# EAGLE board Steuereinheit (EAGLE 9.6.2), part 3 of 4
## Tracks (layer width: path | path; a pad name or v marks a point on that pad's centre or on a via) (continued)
N$83  (via drill 0.35) (continued)
  Top 0.152: v113.72,92.33 112.47,92.33 110.52,90.37 110.52,89.66 PC_JK6.4 | v136.12,95.17 136.12,94.64 137.9,92.86 140.03,92.86 142.16,95 142.16,95.71 PC_AN10.10
  Route2 0.152: v113.72,92.33 114.25,92.33 117.09,95.17 v136.12,95.17
N$84  (via drill 0.35)
  Top 0.152: v115.67,97.49 115.67,95.88 PC_JK6.9 | v115.67,114.02 132.56,114.02 134.16,112.42 134.16,100.86 136.83,98.2 139.68,98.2 140.92,96.95 140.92,95.88 PC_AN10.11
  Bottom 0.152: v115.67,114.02 v115.67,97.49
N$85  (via drill 0.35)
  Top 0.152: PC_JK6.12 111.76,94.64 113,93.4 117.8,93.4 v118.16,93.75 | v135.94,79.17 135.94,77.57 136.65,76.86 138.96,76.86 139.68,77.57 139.68,78.1 PC_AN11.3
  Route15 0.152: v118.16,93.75 122.25,93.75 126.16,89.84 128.65,89.84 135.94,82.55 v135.94,79.17
N$86  (via drill 0.35)
  Top 0.152: v118.16,77.04 117.98,76.86 114.96,76.86 114.43,77.39 114.43,78.1 PC_JK7.7 | v140.74,79.88 140.74,78.46 140.92,78.28 PC_AN11.4
  Route15 0.152: v118.16,77.04 121.72,77.04 122.78,78.1 138.96,78.1 v140.74,79.88
N$87  (via drill 0.35)
  Top 0.152: v122.25,83.97 118.52,83.97 116.38,81.84 112.29,81.84 110.52,80.06 110.52,78.28 PC_JK7.4 | v143.05,82.73 142.34,83.44 142.34,84.33 PC_AN11.10
  Route15 0.152: v122.25,83.97 128.65,83.97 134.16,78.46 136.47,78.46 140.03,82.02 142.34,82.02 v143.05,82.73
N$88  (via drill 0.35)
  Top 0.152: v146.43,96.06 145.01,97.49 143.76,97.49 142.16,99.09 142.16,101.04 PC_AN5.5 | v146.43,70.28 145.9,70.28 143.59,67.97 143.59,66.9 PC_NO1.6
  Bottom 0.152: v146.43,70.28 v146.43,96.06
N$89  (via drill 0.35)
  Top 0.152: v77.62,37.39 76.02,35.79 72.11,35.79 69.98,37.92 69.98,38.63 BR_NO2.14 | v77.27,50.55 76.38,50.55 75.49,51.44 73.18,51.44 72.47,50.72 72.47,50.19 BR_AN1.10 | v87.4,48.41 87.58,48.59 87.58,50.01 BR_JK1.10
  Route15 0.152: v87.4,48.41 86.69,49.12 78.69,49.12 v77.27,50.55
  Bottom 0.152: v77.62,37.39 77.62,40.59 77.98,40.95 77.98,49.84 v77.27,50.55
N$90
  Top 0.152: BR_OR2.4 57.17,66.9 57.17,69.75 59.66,72.24 59.66,72.77 BR_OR2.9
N$91  (via drill 0.35)
  Top 0.152: v125.09,88.06 124.21,88.06 123.32,88.95 123.32,89.48 PC_AN6.1 | v144.3,74.73 144.3,73.3 144.65,72.95 PC_NO1.10
  Route2 0.152: v125.09,88.06 126.34,88.06 126.69,88.42 129.72,88.42 142.7,75.44 143.59,75.44 v144.3,74.73
N$92
  Top 0.152: BR_OR2.3 55.93,66.73 55.93,66.02 58.24,63.7 60.38,63.7 61.62,64.95 61.62,72.24 61.09,72.77 BR_OR2.8
N$93  (via drill 0.35)
  Top 0.152: v135.94,93.22 133.45,95.71 130.96,95.71 PC_AN6.8 | v144.12,71.35 143.23,71.35 142.34,72.24 142.34,72.77 PC_NO1.12
  Route2 0.152: v135.94,93.22 138.61,93.22 139.14,92.69 140.03,92.69 145.36,87.35 145.36,72.59 v144.12,71.35
N$94  (via drill 0.35)
  Top 0.152: v35.84,43.43 33.88,41.48 31.04,41.48 29.26,43.26 29.26,43.79 BR_OR1.3 | v72.82,48.41 72.82,47.88 73.71,46.99 74.42,46.99 74.78,47.35 74.78,50.01 BR_AN1.8
  Route2 0.152: v35.84,43.43 35.84,44.68 42.06,50.9 60.73,50.9 63.22,48.41 v72.82,48.41
N$95
  Top 0.152: PC_NO1.15 138.43,73.48 136.83,75.08 130.78,75.08 130.43,75.44 127.23,75.44 127.05,75.62 125.09,75.62 123.32,77.39 123.32,78.1 PC_AN7.1
N$96  (via drill 0.35)
  Top 0.152: v83.67,20.14 83.67,18.54 BR_AN3.4 | v56.29,68.5 54.51,70.28 54.33,70.28 53.98,70.64 53.98,71.7 54.51,72.24 54.51,72.77 BR_OR2.13
  Route15 0.152: v83.67,20.14 83.67,20.68 72.82,31.52 70.69,31.52 61.09,41.12 57.71,41.12 v55.75,39.17
  Bottom 0.152: v55.75,39.17 55.22,39.7 55.22,67.44 v56.29,68.5
N$97  (via drill 0.35)
  Top 0.152: PC_NO2.2 138.43,54.63 137.72,53.92 136.65,53.92 v133.99,56.59 | v132.92,82.37 130.96,84.33 PC_AN7.8
  Bottom 0.152: v133.99,56.59 133.99,81.31 v132.92,82.37
N$98  (via drill 0.35)
  Top 0.152: v72.11,40.59 69.98,40.59 68.73,39.34 68.73,38.63 BR_NO2.15 | v86.33,48.41 86.33,50.01 BR_JK1.11
  Route2 0.152: v72.11,40.59 79.58,48.06 85.98,48.06 v86.33,48.41
N$99  (via drill 0.35)
  Top 0.152: v131.5,59.26 134.16,59.26 135.23,58.19 139.32,58.19 140.92,56.59 140.92,55.35 PC_NO2.4 | v125.27,64.77 124.56,64.77 123.32,66.02 123.32,66.73 PC_AN8.1
  Route2 0.152: v131.5,59.26 130.78,59.26 v125.27,64.77
N$100  (via drill 0.35)
  Top 0.152: BR_AN3.5 85.09,17.83 88.65,14.28 92.73,14.28 | 92.73,14.28 94.16,14.28 97.71,17.83 | 97.71,17.83 97.71,18.36 BR_AN4.5 97.71,17.83 | v92.73,15.34 92.73,18.36 BR_AN4.1 | 92.73,14.28 v92.73,13.92 | 97.71,17.83 98.42,17.12 100.91,17.12 101.09,17.3 101.09,19.96 100.38,20.68 100.38,24.59 BR_AN4.8 100.2,24.77 100.2,25.48 99.67,26.01 95.94,26.01 95.4,25.48 95.4,24.77 BR_AN4.12 95.4,24.59 95.4,23.52 95.58,23.34 95.58,22.63 95.05,22.1 93.09,22.1 91.14,24.05 87.58,24.05 | v80.64,20.14 80.11,19.61 80.11,18.54 BR_AN3.1 | v80.64,22.63 81.18,22.63 82.42,23.88 | 82.42,23.88 82.42,24.59 BR_AN3.12 82.42,23.88 | 87.58,24.05 87.58,24.59 BR_AN3.8 87.58,24.05 | 87.58,24.05 85.8,22.28 84.02,22.28 82.42,23.88 | v135.23,80.59 138.07,80.59 140.92,83.44 140.92,84.33 PC_AN11.11
  Route2 0.152: v135.23,80.59 134.7,80.59 126.16,72.06 124.21,72.06 109.8,57.66 109.27,57.66 92.56,40.95 92.56,37.92 92.02,37.39 92.02,35.61 84.56,28.14 84.56,26.19 81,22.63 v80.64,22.63
  Bottom 0.152: v92.73,13.92 v92.73,15.34 | v80.64,22.63 v80.64,20.14
N$101  (via drill 0.35)
  Top 0.152: v146.79,57.3 146.79,54.1 146.61,53.92 144.3,53.92 143.59,54.63 143.59,55.35 PC_NO2.6 | v144.3,69.75 133.99,69.75 PC_AN8.8
  Bottom 0.152: v146.79,57.3 144.3,59.79 v144.3,69.75
N$102  (via drill 0.35)
  Top 0.152: v79.22,26.19 77.8,27.61 71.58,27.61 70.87,26.9 70.16,26.9 68.73,25.48 68.73,24.77 BR_OR4.13 | v88.29,22.99 91.67,22.99 92.91,21.74 95.4,21.74 96.47,22.81 96.47,24.59 BR_AN4.11
  Route2 0.152: v88.29,22.99 v85.45,22.99
  Route15 0.152: v79.22,26.19 81.36,26.19 84.56,22.99 v85.45,22.99
N$103  (via drill 0.35)
  Top 0.152: v149.28,91.62 150.17,90.73 150.17,68.33 144.83,62.99 144.83,61.57 PC_NO2.10 | v122.25,100.51 122.61,100.51 123.14,101.04 PC_AN9.1
  Route2 0.152: v149.28,91.62 146.25,91.62 144.65,93.22 139.14,93.22 131.85,100.51 v122.25,100.51
N$104  (via drill 0.35)
  Top 0.152: v81.18,14.45 81,14.28 73.71,14.28 72.64,15.34 70.51,15.34 68.73,17.12 68.73,18.36 BR_OR4.2 | v97.89,22.81 97.89,24.59 BR_AN4.10
  Bottom 0.152: v81.18,14.45 81.53,14.1 81.53,10.36 82.25,9.65 92.02,9.65 92.02,15.7 95.76,19.43 97.89,19.43 v97.89,22.81
N$105  (via drill 0.35)
  Top 0.152: v138.79,63.35 141.1,63.35 142.16,62.28 142.16,61.57 PC_NO2.12 | v132.56,106.38 131.67,106.38 130.96,107.09 PC_AN9.8
  Bottom 0.152: v138.79,63.35 138.79,82.02 138.43,82.37 138.43,103 138.79,103.35 138.79,104.06 136.47,106.38 v132.56,106.38
N$106
  Top 0.152: BR_OR4.6 73.71,18.54 73.71,19.61 75.49,21.39 80.29,21.39 80.47,21.21 89.89,21.21 92.02,19.07 92.02,14.99 92.38,14.63 93.27,14.63 96.47,17.83 96.47,18.36 BR_AN4.4
N$107  (via drill 0.35)
  Top 0.152: PC_NO2.15 138.43,60.86 v137.36,59.79 | v137.36,87.88 137.36,89.31 137.19,89.48 PC_AN10.1
  Bottom 0.152: v137.36,87.88 v137.36,59.79
N$108  (via drill 0.35)
  Top 0.152: v78.69,24.23 78.69,23.52 80.64,21.57 90.07,21.57 90.6,21.03 94.34,21.03 95.22,20.14 95.22,18.54 BR_AN4.3 | v75.31,22.99 74.78,22.99 73.71,24.05 73.71,24.59 BR_OR4.9
  Route2 0.152: v78.69,24.23 76.56,24.23 v75.31,22.99
N$109  (via drill 0.35)
  Top 0.152: BR_NO4.2 40.64,65.3 v40.82,65.13 | v141.28,98.55 142.16,98.55 143.59,97.13 144.12,97.13 144.65,96.6 144.65,95.88 PC_AN10.8
  Route15 0.152: v40.46,99.09 41.17,99.09 47.75,105.66 53.98,105.66 67.13,118.82 119.05,118.82 134.52,103.35 136.47,103.35 v141.28,98.55
  Bottom 0.152: v40.82,65.13 40.82,98.73 v40.46,99.09
N$110  (via drill 0.35)
  Top 0.152: v16.46,40.59 16.46,43.79 BR_NO3.6 | v96.29,40.23 98.07,40.23 98.96,39.34 98.96,38.63 BR_JK6.11
  Route2 0.152: v77.27,33.66 77.27,34.19 84.2,41.12 86.69,41.12 87.58,42.01 v89.71,42.01
  Route15 0.152: v16.46,40.59 16.46,35.43 15.75,34.72 15.75,34.01 16.64,33.12 31.75,33.12 40.46,41.83 57.35,41.83 57.71,42.19 63.4,42.19 71.22,34.37 71.22,33.83 71.58,33.48 77.09,33.48 v77.27,33.66 | v89.71,42.01 94.51,42.01 v96.29,40.23
N$111  (via drill 0.35)
  Top 0.152: v46.15,70.46 43.31,67.62 43.31,66.9 BR_NO4.4 | v136.65,79.88 136.65,78.64 137.01,78.28 PC_AN11.1
  Route15 0.152: v46.15,70.46 46.15,80.95 50.77,85.57 50.77,101.04 51.13,101.4 51.84,101.4 52.55,102.11 64.47,102.11 70.51,108.15 92.38,108.15 95.4,105.13 119.76,105.13 136.65,88.24 136.65,86.28 139.85,83.08 139.85,82.37 137.36,79.88 v136.65,79.88
N$112
  Top 0.152: BR_OR1.4 30.51,43.97 30.51,46.99 32.99,49.48 32.99,50.01 BR_OR1.9
N$113  (via drill 0.35)
  Top 0.152: v46.51,68.5 45.8,67.79 45.8,66.9 BR_NO4.6 | v49.89,96.95 52.73,96.95 54.15,98.37 54.15,99.09 55.04,99.97 57,99.97 57.89,100.86 60.55,100.86 v62.51,102.82 | v144.3,86.11 144.3,84.86 144.65,84.51 PC_AN11.8
  Route15 0.152: v62.51,102.82 63.22,102.82 70.69,110.29 85.45,110.29 85.8,110.64 90.42,110.64 94.16,106.91 118.69,106.91 137.01,88.59 141.81,88.59 v144.3,86.11
  Bottom 0.152: v46.51,68.5 46.86,68.86 46.86,74.91 46.51,75.26 46.51,81.31 49.89,84.68 v49.89,96.95
N$114  (via drill 0.35)
  Top 0.152: v81.89,76.68 75.49,76.68 74.07,75.26 66.42,75.26 65.71,74.55 63.75,74.55 63.58,74.73 61.8,74.73 60.91,75.62 58.42,75.62 57.89,75.08 57.35,75.08 55.93,73.66 55.93,72.95 BR_OR2.12 | v123.5,20.14 123.5,18.72 123.32,18.54 BR_AN2.4
  Route2 0.152: v82.07,26.54 78.51,22.99 77.62,22.99 77.27,22.63 77.27,21.92 77.62,21.57 81.89,21.57 84.2,23.88 89.36,23.88 95.4,17.83 115.14,17.83 118.69,21.39 120.29,21.39 122.25,23.34 122.78,23.34 123.14,23.7 123.85,23.7 124.21,23.34 124.21,20.85 v123.5,20.14
  Bottom 0.152: v81.89,76.68 81.89,78.46 81.53,78.82 80.29,78.82 80.29,31.52 82.07,29.74 v82.07,26.54
N$115  (via drill 0.35)
  Top 0.152: BR_JK3.13 126.34,51.26 126.34,49.48 125.09,48.23 BR_JK3.3 125.09,44.5 126.16,43.43 v126.87,43.43 | BR_JK4.13 140.39,51.26 140.39,49.3 139.14,48.06 139.14,45.21 BR_JK4.3 138.96,45.03 138.96,44.5 138.25,43.79 137.9,43.79 136.83,42.72 130.25,42.72 129.54,43.43 v128.65,43.43
  Route2 0.152: v128.65,43.43 v126.87,43.43
N$116  (via drill 0.35)
  Top 0.152: v76.02,22.1 76.02,25.83 74.6,27.25 71.75,27.25 69.98,25.48 69.98,24.77 BR_OR4.12 | v123.5,22.99 124.38,23.88 124.38,24.59 BR_AN2.10
  Route2 0.152: v76.02,22.1 76.02,21.21 80.47,16.76 104.29,16.76 105,17.48 116.92,17.48 122.43,22.99 v123.5,22.99
N$117  (via drill 0.35)
  Top 0.152: BR_OR4.1 67.31,16.41 68.73,14.99 71.75,14.99 73,13.74 83.49,13.74 v88.47,8.76 | v125.09,22.99 124.38,22.28 123.14,22.28 122.78,22.63 122.78,24.23 123.14,24.59 BR_AN2.11
  Route15 0.152: v88.47,8.76 108.91,8.76 119.58,19.43 121.36,19.43 124.92,22.99 v125.09,22.99
N$118  (via drill 0.35)
  Top 0.152: v78.51,17.12 73.18,17.12 72.47,17.83 72.47,18.36 BR_OR4.5 | v118.34,17.12 121.18,17.12 121.89,17.83 121.89,18.36 BR_AN2.3
  Route2 0.152: v78.51,17.12 79.58,17.12 80.29,16.41 104.47,16.41 105.18,17.12 v118.34,17.12
N$119  (via drill 0.35)
  Top 0.152: v74.24,26.54 74.78,26.01 74.78,24.77 BR_OR4.8 | v71.04,45.57 71.04,50.01 BR_AN1.11
  Route2 0.152: v74.24,26.54 74.24,30.81 71.04,34.01 v71.04,45.57
N$120  (via drill 0.35)
  Top 0.152: v61.98,50.72 61.98,48.95 60.02,46.99 58.24,46.99 55.93,49.3 55.93,50.01 BR_AA2.12 | v62.15,59.44 62.15,62.28 61.44,62.99 56.82,62.99 55.93,62.1 55.93,61.57 BR_AA3.12 | v38.68,52.15 40.46,52.15 41.88,50.72 41.88,50.19 BR_AA1.12 | v38.68,57.66 38.68,58.73 38.86,58.9 | 38.86,58.9 39.04,59.08 40.11,59.08 41.88,60.86 41.88,61.39 BR_AA4.12 | 38.86,58.9 38.33,59.44 38.33,67.79 39.75,69.22 43.84,69.22 46.86,72.24 46.86,72.77 BR_NO4.10
  Route15 0.152: v62.15,59.44 52.38,59.44 50.6,57.66 v38.68,57.66
  Bottom 0.152: v61.98,50.72 62.15,50.9 v62.15,59.44 | v38.68,57.66 v38.68,52.15
N$121  (via drill 0.35)
  Top 0.152: 57.17,52.86 57.17,55.35 BR_AA3.4 | 57.17,52.86 57.17,50.19 BR_AA2.11 | v40.82,45.57 42.24,45.57 43.13,44.68 43.13,43.97 BR_AA1.4 | v40.82,63.7 41.53,63.7 43.13,62.1 43.13,61.57 BR_AA4.11 | v39.04,70.1 40.11,71.17 43.31,71.17 44.37,72.24 44.37,72.77 BR_NO4.12 | v53.44,52.86 57.17,52.86
  Route2 0.152: v39.04,70.1 39.04,65.48 v40.82,63.7
  Route15 0.152: v53.44,52.86 49.71,52.86 42.42,45.57 v40.82,45.57
  Bottom 0.152: v40.82,45.57 40.82,56.41 40.46,56.77 40.46,63.35 v40.82,63.7
N$122  (via drill 0.35)
  Top 0.152: 49,41.83 54.51,41.83 55.75,43.08 55.75,43.79 BR_AA2.3 | 49,41.83 43.31,41.83 42.06,43.08 42.06,43.79 BR_AA1.3 | v49,49.12 48.11,48.23 45.62,48.23 44.55,49.3 44.55,50.01 BR_AA1.10 | 49,41.83 v49,44.14 | 44.55,60.68 44.55,61.39 BR_AA4.10 44.55,60.68 | 44.55,60.68 45.62,59.61 v46.51,59.61 | BR_NO4.15 40.64,73.48 39.57,74.55 v39.39,74.55 | v39.39,58.37 42.24,58.37 44.55,60.68
  Bottom 0.152: v49,49.12 v49,44.14 49,38.1 46.86,38.1 46.51,38.46 v46.51,59.61 | v39.39,74.55 39.75,74.19 39.75,58.73 v39.39,58.37
N$123  (via drill 0.35)
  Top 0.152: v39.39,45.57 39.57,45.57 40.64,44.5 BR_AA1.2 40.64,43.08 42.42,41.3 52.2,41.3 v52.38,41.12 | v39.39,56.95 39.75,56.95 40.64,56.06 BR_AA4.2 | v52.38,42.55 53.8,42.55 54.51,43.26 54.51,43.79 BR_AA2.2 | v52.73,53.57 53.44,53.57 54.51,54.63 54.51,55.35 BR_AA3.2 | v49.53,50.01 48.82,50.01 47.4,48.59 46.51,48.59 45.8,49.3 45.8,50.01 BR_AA1.9 | 61.27,59.26 59.84,60.68 59.84,61.39 BR_AA3.9 | 61.27,59.26 63.04,57.48 63.04,47.52 62.86,47.35 62.86,42.72 63.58,42.01 63.58,39.17 64.29,38.46 64.29,33.66 66.95,30.99 67.67,30.99 68.56,31.88 68.56,32.41 BR_NO2.2 | v59.66,47.7 59.66,50.01 BR_AA2.9 | v59.66,57.48 61.27,59.08 61.27,59.26
  Route15 0.152: v49.53,50.01 49.89,50.01 52.2,47.7 v59.66,47.7
  Bottom 0.152: v39.39,56.95 v39.39,45.57 | v52.73,53.57 52.73,50.01 | 52.73,50.01 52.73,42.9 v52.38,42.55 v52.38,41.12 | 52.73,50.01 v49.53,50.01 | v59.66,57.48 v59.66,47.7
N$124  (via drill 0.35)
  Top 0.152: v18.24,47.7 17.88,48.06 17.88,50.01 BR_NO3.10 | v93.45,30.81 94.16,30.81 95.05,29.92 97.18,29.92 97.71,30.45 97.71,32.41 BR_JK6.5
  Route2 0.152: v66.24,60.86 81.53,60.86 90.96,51.44 v91.85,51.44
  Route15 0.152: v18.24,47.7 18.95,47.7 23.93,52.68 26.59,52.68 32.99,59.08 44.91,59.08 46.68,60.86 v66.24,60.86
  Bottom 0.152: v91.85,51.44 92.2,51.08 92.2,32.05 v93.45,30.81
N$125  (via drill 0.35)
  Top 0.152: v62.15,37.92 58.6,41.48 56.46,41.48 54.86,39.88 42.6,39.88 39.39,43.08 39.39,43.79 BR_AA1.1 | v65.71,53.39 65.71,55.7 66.78,56.77 67.84,56.77 68.56,56.06 68.56,55.35 BR_AN5.2 | v107.31,28.85 108.2,28.85 109.27,29.92 111.58,29.92 112.29,29.21 116.03,29.21 117.45,30.63 117.45,32.23 114.96,34.72 114.96,38.63 BR_OR7.8
  Route15 0.152: v107.31,28.85 107.31,30.1 102.69,34.72 102.69,35.43 90.42,47.7 75.13,47.7 72.11,50.72 68.38,50.72 v65.71,53.39
  Bottom 0.152: v62.15,37.92 64.64,40.41 64.64,52.32 v65.71,53.39
N$126  (via drill 0.35)
  Top 0.152: BR_AA1.13 40.64,50.72 39.93,51.44 38.33,51.44 37.97,51.08 37.26,51.08 36.91,51.44 36.91,52.15 37.62,52.86 48.11,52.86 49.53,54.28 v49.53,56.95 | v73.53,57.3 73.53,55.35 BR_AN5.6
  Route2 0.152: v49.53,56.95 53.09,56.95 53.8,56.24 54.86,56.24 55.22,55.88 72.11,55.88 v73.53,57.3
N$127  (via drill 0.35)
  Top 0.152: BR_AN5.1 67.31,54.63 68.38,53.57 69.09,53.57 69.44,53.21 v69.44,52.15 | 69.44,62.99 69.44,61.92 69.8,61.57 BR_AN5.12 | v69.62,34.37 69.8,34.37 71.04,33.12 71.04,32.59 BR_NO2.4 | v71.04,53.39 72.29,54.63 72.29,55.35 BR_AN5.5 | PC_AN4.1 106.07,55.35 v105.18,56.24 | 69.44,62.99 74.07,62.99 74.78,62.28 74.78,61.57 BR_AN5.8 | 69.44,62.99 v69.44,63.17
  Route2 0.152: v69.44,52.15 70.69,53.39 v71.04,53.39 71.75,52.68 76.2,52.68 78.16,50.72 93.8,50.72 99.31,56.24 v105.18,56.24
  Bottom 0.152: v69.44,63.17 69.09,62.81 69.09,57.48 69.44,57.12 v69.44,52.15 69.09,51.79 69.09,34.9 v69.62,34.37
N$128  (via drill 0.35)
  Top 0.152: 76.56,58.01 79.22,58.01 81.18,56.06 81.18,55.35 BR_OR5.2 | 76.56,58.01 73.18,58.01 71.22,56.06 71.22,55.35 BR_AN5.4 | v76.91,40.23 76.91,40.95 76.38,41.48 73.71,41.48 72.47,42.72 72.47,43.79 BR_AN1.5 | 76.56,58.01 v76.56,54.28
  Bottom 0.152: v76.91,40.23 77.09,40.41 77.09,49.66 76.56,50.19 v76.56,54.28
N$129
  Top 0.152: BR_OR5.1 79.93,55.17 78.51,55.17 76.02,52.68 70.69,52.68 69.98,53.39 69.98,55.35 BR_AN5.3
N$130  (via drill 0.35)
  Top 0.152: v70.16,42.19 69.98,42.37 69.98,43.79 BR_AN1.3 | v101.98,35.08 106.6,35.08 108.56,33.12 108.56,32.59 BR_OR7.2
  Route15 0.152: v70.16,42.19 71.58,42.19 71.75,42.37 72.47,42.37 74.24,40.59 74.24,40.41 76.56,38.1 78.69,38.1 81.18,35.61 98.42,35.61 99.49,34.54 101.45,34.54 v101.98,35.08
N$131  (via drill 0.35)
  Top 0.152: v51.31,43.26 51.84,43.79 53.26,43.79 BR_AA2.1 | v73.18,59.61 73.18,61.04 73.53,61.39 BR_AN5.9
  Route2 0.152: v54.15,56.95 54.69,56.95 55.4,56.24 68.38,56.24 71.22,59.08 72.64,59.08 v73.18,59.61
  Bottom 0.152: v51.31,43.26 51.31,40.77 51.66,40.41 54.15,40.41 v54.15,56.95
N$132  (via drill 0.35)
  Top 0.152: v37.62,42.55 36.55,42.55 35.13,41.12 30.86,41.12 30.33,41.66 26.95,41.66 25.88,42.72 25.88,45.39 27.84,47.35 27.84,50.01 BR_OR1.13 | v65.35,45.92 67.31,43.97 BR_AN1.1 | v68.02,59.44 68.38,59.08 71.75,59.08 72.29,59.61 72.29,61.39 BR_AN5.10
  Route2 0.152: v37.62,42.55 46.33,42.55 48.64,44.86 64.29,44.86 v65.35,45.92
  Bottom 0.152: v68.02,59.44 66.42,57.84 66.42,46.99 v65.35,45.92
N$133  (via drill 0.35)
  Top 0.152: v72.11,41.66 71.22,42.55 71.22,43.79 BR_AN1.4 | v102.34,34.01 105.89,34.01 107.31,32.59 BR_OR7.1
  Route15 0.152: v72.11,41.66 77.44,36.32 78.51,36.32 80.82,34.01 v102.34,34.01
N$134  (via drill 0.35)
  Top 0.152: v38.33,49.66 38.15,49.66 36.37,51.44 29.97,51.44 29.26,50.72 29.26,50.19 BR_OR1.12 | v81,53.75 81.53,53.75 82.42,54.63 82.42,55.17 BR_OR5.3
  Route15 0.152: v38.33,49.66 43.84,49.66 47.57,53.39 51.49,53.39 52.38,54.28 65.89,54.28 69.09,51.08 71.22,51.08 73,52.86 73,54.1 73.89,54.99 79.76,54.99 v81,53.75
N$135  (via drill 0.35)
  Top 0.152: v54.15,58.73 53.44,58.01 53.44,55.35 BR_AA3.1 | v73.18,68.5 73.18,68.15 72.47,67.44 72.47,66.9 BR_AN6.5 | v106.07,40.95 107.31,42.19 115.67,42.19 116.38,42.9 116.38,45.03 115.67,45.75 115.67,50.01 BR_OR6.8
  Route2 0.152: v54.15,58.73 55.4,58.73 67.13,70.46 67.13,70.81 67.49,71.17 68.2,71.17 70.16,69.22 72.47,69.22 v73.18,68.5
  Route15 0.152: v106.07,40.95 101.8,40.95 92.38,50.37 78.51,50.37 75.84,53.04 74.42,53.04 v73.71,53.75
  Bottom 0.152: v73.71,53.75 74.07,54.1 74.07,56.59 74.42,56.95 74.42,67.26 v73.18,68.5
N$136  (via drill 0.35)
  Top 0.152: v52.38,60.15 53.98,60.15 54.51,60.68 54.51,61.39 BR_AA3.13 | v75.84,71.17 75.84,71.88 74.95,72.77 BR_AN6.8 | v114.96,47.52 114.43,48.06 114.43,50.01 BR_OR6.9
  Route2 0.152: v52.38,60.15 53.62,60.15 65.18,71.7 68.73,71.7 68.91,71.88 71.93,71.88 73.36,70.46 75.13,70.46 v75.84,71.17 | v114.96,47.52 103.05,47.52 102.87,47.7 102.16,47.7 100.91,46.46 v99.67,46.46
  Route15 0.152: v99.67,46.46 99.14,46.46 97.54,48.06 97.54,48.23 95.05,50.72 78.87,50.72 75.84,53.75 v75.67,53.75
  Bottom 0.152: v75.67,53.75 75.84,53.92 v75.84,71.17
N$137  (via drill 0.35)
  Top 0.152: v36.91,53.21 37.97,53.21 39.22,54.46 39.22,55.35 BR_AA4.1 | v36.91,47.17 48.11,47.17 50.24,49.3 50.24,62.46 51.31,63.52 56.29,63.52 56.46,63.35 63.22,63.35 65,65.13 65,73.3 | 65,73.3 66.6,74.91 68.56,74.91 69.8,73.66 69.8,72.95 BR_AN6.12 | v108.91,51.79 109.45,51.79 110.34,50.9 110.34,50.19 BR_OR6.12 | 65,73.3 v65.53,73.3
  Route15 0.152: v108.38,58.55 108.38,59.08 106.07,61.39 105.54,61.39 104.65,62.28 101.09,62.28 99.85,63.52 97.71,63.52 97.36,63.17 96.65,63.17 96.29,63.52 96.29,65.13 92.91,68.5 89.18,68.5 84.38,73.3 v65.53,73.3
  Bottom 0.152: v36.91,47.17 v36.91,53.21 | v108.91,51.79 108.38,52.32 v108.38,58.55
N$138  (via drill 0.35)
  Top 0.152: BR_AA4.13 40.64,60.86 39.57,59.79 v39.04,59.79 | v66.06,66.19 66.78,66.19 67.31,66.73 BR_AN6.1 | v106.96,49.12 107.49,48.59 108.38,48.59 109.09,49.3 109.09,50.01 BR_OR6.13
  Route2 0.152: v39.04,59.79 45.26,59.79 47.04,58.01 55.75,58.01 63.93,66.19 v66.06,66.19 68.38,66.19 72.47,62.1 93.98,62.1 99.14,56.95 v106.96,56.95
  Bottom 0.152: v106.96,56.95 v106.96,49.12
N$139
  Top 0.152: BR_AN6.4 71.22,66.73 71.22,66.02 73,64.24 81.18,64.24 81.53,64.59 87.05,64.59 88.47,63.17 88.47,60.5 85.98,58.01 85.8,58.01 85.27,57.48 85.27,55.35 BR_OR5.5
N$140  (via drill 0.35)
  Top 0.152: v86.16,57.3 86.33,57.12 86.33,55.35 BR_OR5.6 | v77.27,69.57 76.73,69.57 76.2,70.1 73.71,70.1 72.47,71.35 72.47,72.77 BR_AN6.10
  Route15 0.152: v86.16,57.3 77.27,66.19 v77.27,69.57
N$141
  Top 0.152: BR_OR5.12 82.6,61.39 82.6,57.12 83.67,56.06 83.67,55.35 BR_OR5.4
N$142
  Top 0.152: BR_OR5.13 81.36,61.57 81.36,62.28 82.07,62.99 84.2,62.99 85.09,62.1 85.09,61.57 BR_OR5.10
N$143  (via drill 0.35)
  Top 0.152: v67.84,70.46 69.62,70.46 71.04,71.88 71.04,72.77 BR_AN6.11 | v87.4,63.17 87.4,61.75 87.58,61.57 BR_OR5.8
  Route2 0.152: v67.84,70.46 67.84,69.93 74.95,62.81 85.62,62.81 85.98,62.46 86.69,62.46 v87.4,63.17
N$144  (via drill 0.35)
  Top 0.152: v71.04,68.5 70.87,68.5 69.98,67.62 69.98,66.9 BR_AN6.3 | v86.33,63.17 86.33,61.57 BR_OR5.9
  Route2 0.152: v71.04,68.5 73.53,66.02 82.25,66.02 85.09,63.17 v86.33,63.17
N$145  (via drill 0.35)
  Top 0.152: v85.45,59.79 84.91,59.79 83.84,60.86 83.84,61.39 BR_OR5.11 | v85.45,63.88 84.91,63.88 84.56,64.24 81.71,64.24 81.36,63.88 69.09,63.88 68.73,63.52 68.73,61.57 BR_AN5.13
  Bottom 0.152: v85.45,63.88 v85.45,59.79
N$146  (via drill 0.35)
  Top 0.152: v28.91,45.57 28.02,44.68 28.02,43.97 BR_OR1.2 | v71.4,59.79 71.4,61.21 BR_AN5.11
  Route2 0.152: v28.91,45.57 32.64,45.57 36.91,49.84 36.91,52.15 40.64,55.88 54.15,55.88 54.51,55.52 73,55.52 74.42,56.95 74.42,59.97 74.07,60.33 71.93,60.33 v71.4,59.79
N$147
  Top 0.152: BR_OR1.1 26.77,43.97 26.77,45.75 30.33,49.3 30.33,50.01 BR_OR1.11
N$148
  Top 0.152: BR_JK2.5 97.71,43.79 97.71,42.72 96.29,41.3 92.2,41.3 91.14,42.37 91.14,45.75 89.71,47.17 84.73,47.17 82.6,49.3 82.6,50.01 BR_JK1.14
N$149  (via drill 0.35)
  Top 0.152: v16.64,48.23 16.46,48.23 15.39,49.3 15.39,50.01 BR_NO3.12 | v82.07,40.23 85.45,40.23 86.33,39.34 86.33,38.63 BR_JK5.11
  Route2 0.152: v76.56,34.37 76.56,34.72 v82.07,40.23
  Route15 0.152: v16.64,48.23 17.88,46.99 23.22,46.99 30.33,54.1 32.46,54.1 32.99,53.57 32.99,47.35 35.84,44.5 47.57,44.5 48.64,43.43 50.42,43.43 50.95,43.97 63.75,43.97 67.31,40.41 67.31,39.34 71.75,34.9 76.02,34.9 v76.56,34.37
N$150  (via drill 0.35)
  Top 0.152: v82.25,34.72 82.42,34.54 82.42,32.59 BR_JK5.3 | v82.25,36.86 82.6,36.86 83.67,37.92 83.67,38.63 BR_JK5.13 | v93.8,34.72 95.22,33.3 95.22,32.59 BR_JK6.3 | v93.8,36.86 95.4,36.86 96.47,37.92 96.47,38.63 BR_JK6.13 | v111.05,20.14 111.05,18.54 BR_AN7.4
  Route2 0.152: v111.05,20.14 96.47,34.72 v93.8,34.72
  Route15 0.152: v82.25,34.72 88.11,34.72 88.29,34.54 93.62,34.54 v93.8,34.72
  Bottom 0.152: v82.25,36.86 v82.25,34.72 | v93.8,36.86 v93.8,34.72
N$151
  Top 0.152: BR_JK2.2 93.98,45.75 95.22,46.99 97.89,46.99 98.96,48.06 98.96,50.01 BR_JK2.11
N$152  (via drill 0.35)
  Top 0.152: v25.35,40.41 21.97,43.79 21.97,50.55 20.37,52.15 12.9,52.15 11.48,50.72 11.48,50.19 BR_NO3.15 | v47.4,36.68 59.84,36.68 67.84,28.68 83.84,28.68 85.45,30.28 85.45,32.05 85.09,32.41 BR_JK5.5
  Route2 0.152: v25.35,40.41 26.77,40.41 30.51,36.68 v47.4,36.68
N$153  (via drill 0.35)
  Top 0.152: v111.4,48.41 110.52,47.52 110.52,43.97 BR_OR6.3 | v115.49,82.55 115.49,84.33 PC_JK7.9
  Route15 0.152: v111.4,48.41 111.94,48.41 v115.49,51.97
  Bottom 0.152: v115.49,82.55 v115.49,51.97
N$154  (via drill 0.35)
  Top 0.152: v73.71,34.19 73.71,32.59 BR_NO2.6 | v74.07,47.7 74.07,49.66 BR_AN1.9 | PC_JK7.12 111.76,87.53 v111.4,87.88 v106.6,87.88 | v136.65,82.55 137.19,82.55 138.43,83.8 PC_AN11.13
  Route2 0.152: v111.4,87.88 122.07,87.88 123.14,88.95 129.72,88.95 136.12,82.55 v136.65,82.55 | v74.07,47.7 76.2,47.7 77.27,48.77 85.09,48.77 86.16,49.84 94.69,49.84 100.02,55.17 v105.18,55.17
  Bottom 0.152: v73.71,34.19 74.07,34.54 v74.07,47.7 | v105.18,55.17 105.89,55.88 105.89,59.44 105.54,59.79 105.54,80.42 106.6,81.48 v106.6,87.88
N$155  (via drill 0.35)
  Top 0.152: BR_OR1.10 31.75,48.95 29.08,46.28 28.55,46.28 v27.84,45.57 | v75.13,34.19 75.13,32.77 74.95,32.59 BR_NO2.7
  Route2 0.152: v27.84,45.57 30.51,42.9 33.88,42.9 36.37,40.41 47.04,40.41 49.35,38.1 58.78,38.1 64.64,32.23 67.49,32.23 73.89,25.83 74.6,25.83 74.95,26.19 74.95,29.92 74.6,30.28 74.6,33.48 75.13,34.01 v75.13,34.19
N$156  (via drill 0.35)
  Top 0.152: BR_JK8.11 142.88,41.48 v143.05,41.66 | v101.98,58.9 100.56,57.48 100.38,57.48 99.14,56.24 99.14,55.35 BR_NO1.6
  Route15 0.152: v143.05,41.66 143.05,38.99 143.41,38.63 143.41,37.92 143.05,37.57 136.3,37.57 129.01,44.86 106.25,44.86 v102.69,48.41
  Bottom 0.152: v102.69,48.41 101.98,49.12 v101.98,58.9
N$157  (via drill 0.35)
  Top 0.152: v142.7,38.28 141.63,37.21 141.63,33.83 BR_JK8.5 | v100.02,59.79 100.02,61.21 100.2,61.39 BR_NO1.10
  Route15 0.152: v142.7,38.28 141.1,38.28 122.96,56.41 111.58,56.41 110.16,57.84 101.98,57.84 v100.02,59.79
N$158  (via drill 0.35)
  Top 0.152: v101.09,64.41 100.02,64.41 97.89,62.28 97.89,61.57 BR_NO1.12 | v124.56,37.39 127.05,37.39 128.83,39.17 128.83,39.88 BR_JK7.11
  Route2 0.152: v102.69,49.48 103.4,49.48 104.83,48.06 109.98,48.06 111.05,49.12 119.58,49.12 125.09,43.61 125.09,37.92 v124.56,37.39
  Bottom 0.152: v101.09,64.41 101.45,64.06 102.69,64.06 v102.69,49.48
N$159  (via drill 0.35)
  Top 0.152: v37.62,45.39 33.88,45.39 33.17,44.68 33.17,43.97 BR_OR1.6 | v79.22,46.1 79.22,47.35 81.18,49.3 81.18,50.01 BR_JK1.15 | v99.85,41.83 99.14,42.55 99.14,43.79 BR_JK2.6
  Route15 0.152: v37.62,45.39 38.51,45.39 39.04,44.86 42.6,44.86 49.89,52.15 55.57,52.15 56.46,53.04 65,53.04 71.04,46.99 76.02,46.99 76.2,47.17 78.16,47.17 v79.22,46.1 84.2,46.1 90.78,39.52 97.54,39.52 99.85,37.21 v99.85,35.26
  Bottom 0.152: v99.85,35.26 v99.85,41.83
N$160  (via drill 0.35)
  Top 0.152: v14.68,40.23 14.5,40.23 11.48,43.26 11.48,43.79 BR_NO3.2 | v149.28,27.08 149.28,49.3 145.9,52.68 143.59,52.68 142.88,51.97 BR_JK4.11
  Route2 0.152: v14.68,40.23 15.04,40.23 16.1,41.3 20.37,41.3 26.24,35.43 41,35.43 69.8,6.63 77.44,6.63 82.07,2.01 131.14,2.01 142.16,13.03 148.92,13.03 149.28,13.39 v149.28,27.08
N$161  (via drill 0.35)
  Top 0.152: BR_NO3.4 13.97,42.01 16.1,39.88 16.81,39.88 18.77,41.83 v20.9,41.83 | v89.53,36.86 89.89,36.86 91.31,35.43 91.31,35.26 91.49,35.08 91.49,30.99 92.56,29.92 94.51,29.92 95.94,28.5 105.89,28.5 107.49,30.1 108.91,30.1 109.09,30.28 111.76,30.28 112.47,29.57 115.32,29.57 v116.74,30.99 | v141.1,43.43 141.1,44.68 BR_JK4.5
  Route2 0.152: v20.9,41.83 21.97,41.83 22.33,42.19 26.42,42.19 28.91,39.7 42.42,39.7 44.73,37.39 54.51,37.39 57.17,34.72 60.55,34.72 70.16,25.12 75.67,25.12 87.4,36.86 v89.53,36.86 | v116.74,30.99 119.23,30.99 119.41,30.81 127.41,30.81 140.03,43.43 v141.1,43.43
N$162  (via drill 0.35)
  Top 0.152: v73.36,37.03 73.89,37.03 74.78,37.92 74.78,38.63 BR_NO2.10 | v128.65,49.66 128.65,51.08 BR_JK3.11
  Route2 0.152: v73.36,37.03 73.36,41.3 79.76,47.7 95.76,47.7 v100.56,52.5
  Route15 0.152: v100.56,52.5 101.09,52.5 101.98,53.39 109.09,53.39 111.05,55.35 121.54,55.35 127.23,49.66 v128.65,49.66
N$163  (via drill 0.35)
  Top 0.152: v92.73,29.21 91.14,30.81 91.14,34.9 90.96,35.08 90.96,35.26 90.07,36.14 89.18,36.14 88.82,36.5 85.98,36.5 85.62,36.14 80.29,36.14 78.33,38.1 77.27,38.1 76.91,37.74 76.91,37.39 75.67,36.14 73.18,36.14 72.47,36.86 72.47,38.63 BR_NO2.12 | v122.78,43.26 124.56,43.26 125.09,42.72 127.23,42.72 127.58,43.08 127.58,45.03 BR_JK3.5
  Route2 0.152: v92.73,29.21 92.73,37.03 93.98,38.28 93.98,40.59 95.94,42.55 122.07,42.55 v122.78,43.26
N$164  (via drill 0.35)
  Top 0.152: BR_NO1.15 93.98,59.97 v94.16,59.79 | v126.34,32.05 126.69,32.41 126.87,32.41 127.58,33.12 127.58,33.66 BR_JK7.5
  Route2 0.152: v94.69,40.23 97.18,37.74 120.65,37.74 v126.34,32.05
  Bottom 0.152: v94.16,59.79 94.16,40.77 v94.69,40.23
N$166  (via drill 0.35)
  Top 0.152: BR_JK1.5 85.09,44.5 86.33,45.75 v90.07,45.75 | v92.2,52.86 95.94,52.86 96.47,53.39 96.47,55.35 BR_NO1.4
  Bottom 0.152: v90.07,45.75 90.42,46.1 90.42,58.19 90.96,58.73 92.2,58.73 v92.2,52.86
N$167  (via drill 0.35)
  Top 0.152: v113.18,30.81 112.47,31.52 112.47,32.41 BR_OR7.5 | v113.18,45.57 113.18,50.01 BR_OR6.10
  Bottom 0.152: v113.18,45.57 v113.18,30.81
N$168
  Top 0.152: M_CLK.2 53.09,14.45 53.09,5.38 52.2,4.5 CLKNO.10
N$169
  Top 0.152: SE_BF7.4 55.4,78.46 57.71,78.46 58.6,79.35 SEN7.1
N$170
  Top 0.152: SE_BF6.4 55.4,83.62 57.89,83.62 58.6,84.33 SEN6.1
N$171
  Top 0.152: SE_BF5.4 55.4,88.59 57.71,88.59 58.6,89.48 SEN5.1
N$172
  Top 0.152: SE_BF4.4 55.4,93.75 57.89,93.75 58.6,94.46 SEN4.2
N$173
  Top 0.152: SE_BF3.4 55.4,98.91 57.89,98.91 58.6,99.62 SEN3.2
N$174
  Top 0.152: SE_BF2.4 55.4,103.89 57.71,103.89 58.6,104.78 SEN2.2
N$175
  Top 0.152: SE_BF1.4 55.4,109.04 57.89,109.04 58.6,109.75 SEN1.2
N$176
  Top 0.152: SE_BF0.4 55.4,114.02 57.71,114.02 58.6,114.91 SEN0.2
N$177
  Top 0.152: CLKNO.11 54.69,4.5 57,4.5 CLKNO.12
N$178  (via drill 0.35)
  Top 0.152: v16.99,69.22 19.13,69.22 19.3,69.04 21.44,69.04 SE_CLK.1 | v12.01,69.22 10.24,67.44 10.24,66.9 SE_JK12.1
  Route2 0.152: v12.01,69.22 v16.99,69.22
N$179  (via drill 0.35)
  Top 0.152: v103.4,6.1 103.4,6.63 104.65,7.87 C_P.2 | v57.53,21.39 57.53,18.9 M_NO1.6
  Route2 0.152: v103.4,6.1 103.4,3.96 101.8,2.36 92.56,2.36 81.71,13.21 63.93,13.21 45.26,31.88 45.26,34.19 45.62,34.54 46.33,34.54 57.53,23.34 v57.53,21.39
N$180
  Top 0.152: CLKNO.4 54.69,11.96 54.69,9.47 59.66,4.5 CLKNO.13
N$181
  Top 0.152: 106.07,6.1 107.31,6.1 C_H.1 | 106.07,6.1 104.83,6.1 C_P.1 | 106.07,6.1 106.07,3.96 CHECK.1
N$182
  Top 0.152: MCLKR3.A 29.26,6.45 31.75,6.45 MCLKR2.2
N$183
  Top 0.152: M_NO1.2 52.2,18.36 52.2,17.83 53.62,16.41 54.86,16.41 55.57,15.7 61.98,15.7 63.58,17.3 63.58,26.01 60.73,28.85 60.73,32.05 59.13,33.66 PLR.1 53.62,33.66 50.6,30.63 49,30.63 PLD.A
N$184
  Top 0.152: 47.22,29.39 47.22,32.05 48.82,33.66 PLR.2 | 47.22,29.39 47.22,23.7 45.8,22.28 43.13,22.28 40.11,19.25 40.11,18.54 PL_XR.2 | 47.22,29.39 49.89,29.39 50.95,30.45 58.95,30.45 PLD.C
  Bottom 0.152: PLC.1 62.86,30.63 59.13,30.63 PLD.C
N$185  (via drill 0.35)
  Top 0.152: v60.02,38.99 59.13,39.88 55.4,39.88 55.04,39.52 41.53,39.52 40.11,38.1 40.11,36.14 M_OR1.13 | v62.86,75.97 74.24,75.97 75.31,77.04 81.18,77.04 81.53,77.39 84.73,77.39 87.76,74.37 89.18,74.37 93.45,70.1 101.8,70.1 105.18,66.73 105.18,64.95 106.07,64.06 111.58,64.06 111.76,64.24 113.36,64.24 v113.72,64.59 | v114.78,53.75 112.65,53.75 111.76,54.63 PC_AN4.4
  Bottom 0.152: v60.02,38.99 60.73,39.7 62.15,39.7 62.15,46.99 62.86,47.7 v62.86,75.97 | v113.72,64.59 114.78,63.52 v114.78,53.75
N$186
  Top 0.152: READ.4 134.7,3.96 134.7,8.41 WR_BF0.4 134.7,8.59 135.59,9.47 144.65,9.47 RE_BF0.2
N$187
  Top 0.152: PL_XR.3 41.35,18.54 41.35,19.25 42.95,20.85 54.15,20.85 55.75,19.25 55.75,18.54 M_NO1.5
N$188
  Top 0.152: RE_BF1.2 144.65,14.45 144.3,14.45 143.59,13.74 134.7,13.74 WR_BF1.4 134.52,13.56 133.63,12.68 133.63,5.74 133.45,5.56 133.45,2.54 134.16,1.83 135.05,1.83 137.01,3.79 READ.3
N$189  (via drill 0.35)
  Top 0.152: v42.77,37.74 42.6,37.57 42.6,36.14 M_OR1.11 | v79.93,103.18 85.09,103.18 85.62,102.64 89.18,102.64 92.2,99.62 94.51,99.62 95.22,100.33 95.22,101.04 PC_JK1.3
  Route15 0.152: v42.77,37.74 43.66,37.74 45.8,39.88 55.93,39.88 57.89,41.83 63.22,41.83 70.87,34.19 70.87,33.66 72.29,32.23 78.51,32.23 v79.93,30.81
  Bottom 0.152: v79.93,103.18 v79.93,30.81
N$190  (via drill 0.35)
  Top 0.152: 139.68,18.9 143.59,18.9 144.3,19.61 144.65,19.61 RE_BF2.2 | 139.68,18.9 134.7,18.9 WR_BF2.4 | 139.68,18.9 v139.68,14.45
  Bottom 0.152: v139.68,14.45 139.68,3.96 READ.2
N$191  (via drill 0.35)
  Top 0.152: v45.8,38.81 42.42,38.81 41.35,37.74 41.35,36.14 M_OR1.12 | v113.36,59.79 113.36,61.21 113.18,61.39 PC_AN4.10
  Route2 0.152: v78.51,22.28 79.93,22.28 80.29,21.92 81,21.92 92.38,33.3 92.38,37.21 93.62,38.46 93.62,41.48 99.31,47.17 100.91,47.17 101.98,48.23 101.98,49.84 108.38,56.24 110.34,56.24 113.36,59.26 v113.36,59.79
  Route15 0.152: v45.8,38.81 46.15,38.81 47.57,37.39 59.31,37.39 73,23.7 77.09,23.7 v78.51,22.28
N$192
  Top 0.152: 143.41,23.88 134.7,23.88 WR_BF3.4 | 143.41,23.88 144.3,24.77 RE_BF3.2 | 143.41,23.88 143.41,23.34 145.9,20.85 145.9,20.14 146.25,19.79 146.25,8.59 142.34,4.67 142.34,3.96 READ.1
N$193
  Top 0.152: WR_BF0.2 132.03,9.47 131.67,9.47 127.05,4.85 127.05,3.96 REGISTER.4
N$194
  Top 0.152: WR_BF1.2 132.03,14.45 130.78,14.45 124.74,8.41 124.74,4.14 124.56,3.96 REGISTER.3
N$195
  Top 0.152: WR_BF2.2 132.03,19.61 130.61,19.61 128.12,17.12 128.12,16.41 122.07,10.36 122.07,3.96 REGISTER.2
N$196
  Top 0.152: WR_BF3.2 131.67,24.77 127.76,20.85 127.76,16.59 119.41,8.23 119.41,3.96 REGISTER.1
N$197
  Top 0.152: 132.56,15.52 133.1,14.99 133.1,13.21 132.21,12.32 132.21,10.54 WR_BF0.1 | 132.56,15.52 132.21,15.52 WR_BF1.1 132.56,15.52 | 132.74,20.5 132.21,20.5 WR_BF2.1 | 132.74,20.5 133.1,20.14 133.1,16.05 132.56,15.52 | 132.74,20.5 133.1,20.85 133.1,25.12 132.56,25.65 132.21,25.65 WR_BF3.1
N$198
  Top 0.152: M_OR1.6 45.09,31.34 48.82,35.08 59.13,35.08 61.8,32.41 61.8,28.32 63.93,26.19 63.93,13.74 65.18,12.5 65.18,6.81 66.24,5.74 T1.A1
N$199
  Top 0.152: MCLKR3.S 26.77,3.96 26.77,12.68 MCLKC.1
  Route2 0.152: CLKNO.1 62.15,11.96 61.09,11.96 60.2,11.07 58.95,11.07 58.42,11.61 58.24,11.61 57.71,11.07 28.37,11.07 26.77,12.68 MCLKC.1
N$200  (via drill 0.35)
  Top 0.152: v48.46,92.69 50.42,90.73 50.42,80.24 51.13,79.53 52.55,79.53 SE_BF7.2 | 48.46,104.6 48.46,106.91 48.28,107.09 SE_AN2.8 | 48.46,104.6 v48.46,102.82 | 48.46,104.6 28.73,104.6 28.02,105.31 28.02,107.09 SE_JK11.14
  Bottom 0.152: v48.46,102.82 v48.46,92.69
N$201  (via drill 0.35)
  Top 0.152: v47.4,92.51 50.06,89.84 50.06,78.99 52.38,76.68 53.09,76.68 53.8,77.39 53.8,83.8 53.26,84.33 52.73,84.33 SE_BF6.2 | v47.4,99.44 47.4,100.69 47.04,101.04 SE_AN2.6 46.86,101.22 46.86,101.75 44.37,104.24 34.92,104.24 33.91,103.23 v33.58,103.23 | v26.59,103.53 26.59,101.22 SE_JK11.2
  Route15 0.152: v26.59,103.53 33.27,103.53 v33.58,103.23
  Bottom 0.152: v47.4,99.44 v47.4,92.51
N$202  (via drill 0.35)
  Top 0.152: v49.17,96.24 53.44,96.24 53.8,95.88 53.8,93.4 51.66,91.26 51.66,90.19 52.2,89.66 52.55,89.66 SE_BF5.2 | v28.19,94.11 28.19,95.53 SE_JK10.14
  Route2 0.152: v49.17,96.24 30.33,96.24 v28.19,94.11
N$203  (via drill 0.35)
  Top 0.152: v49.17,94.64 52.55,94.64 SE_BF4.2 | v41.88,94.11 41.88,95.71 SE_AN1.13 | v24.46,90.55 24.99,91.08 25.88,91.08 26.59,90.37 26.59,89.66 SE_JK10.2
  Route2 0.152: v49.17,94.64 42.42,94.64 v41.88,94.11 38.33,90.55 v24.46,90.55
N$204  (via drill 0.35)
  Top 0.152: v49.53,102.82 50.77,101.57 50.77,100.33 51.31,99.8 52.55,99.8 SE_BF3.2 | v34.95,91.26 34.95,82.73 33.71,81.48 29.79,81.48 28.02,83.26 28.02,84.33 SE_JK9.14
  Route15 0.152: v49.53,102.82 48.82,103.53 47.22,103.53 43.31,99.62 43.31,99.09 35.48,91.26 v34.95,91.26
N$205  (via drill 0.35)
  Top 0.152: v41.88,115.62 46.01,115.62 46.55,115.09 52.55,115.09 SE_BF0.2 | v38.33,79.35 38.33,77.39 38.86,76.86 39.93,76.86 40.64,77.57 SE_JK8.2
  Bottom 0.152: v41.88,115.62 38.33,112.06 v38.33,79.35
N$206  (via drill 0.35)
  Top 0.152: v53.26,107.09 53.8,107.62 53.8,109.22 53.26,109.75 52.73,109.75 SE_BF1.2 | v46.86,87.88 44.73,87.88 42.06,85.22 42.06,84.51 SE_JK8.14
  Route2 0.152: v53.26,107.09 53.26,94.82 46.86,88.42 v46.86,87.88
N$207  (via drill 0.35)
  Top 0.152: SE_BF2.2 52.38,104.78 51.66,105.49 v51.66,106.38 | v24.64,76.68 25.7,76.68 26.59,77.57 26.59,78.1 SE_JK9.2
  Route2 0.152: v51.66,106.38 51.66,101.93 50.6,100.86 50.6,95 49,93.4 47.04,93.4 40.46,86.82 36.91,86.82 26.77,76.68 v24.64,76.68
N$208
  Top 0.152: M_NO1.15 52.2,24.59 52.2,23.88 52.91,23.16 56.29,23.16 57,23.88 57,24.59 M_NO1.11
N$209
  Top 0.152: M_NO1.12 55.93,24.77 55.93,25.3 56.64,26.01 58.95,26.01 59.66,25.3 59.66,24.77 M_NO1.9
N$210
  Top 0.152: M_NO1.10 M_NO1.7
N$211
  Top 0.152: CLKNO.2 59.66,12.14 57.17,12.14 CLKNO.3
  Route15 0.152: MCLKR1.1 31.75,9.47 32.82,8.41 53.44,8.41 57,11.96 CLKNO.3
N$212
  Top 0.152: MCLKR2.1 41.88,6.45 41.88,9.47 MCLKR1.2
N$213  (via drill 0.35)
  Top 0.152: v114.61,30.63 113.72,31.52 113.72,32.41 BR_OR7.6 | v114.25,51.79 112.83,51.79 111.76,50.72 BR_OR6.11
  Bottom 0.152: v114.61,30.63 114.25,30.99 v114.25,51.79
N$214
  Top 0.152: MCLKR4.2 72.29,10.9 67.67,10.9 66.42,12.14 T1.A2
N$215
  Top 0.152: BR_OR7.4 111.23,32.59 111.23,35.61 113.54,37.92 113.54,38.63 BR_OR7.9
N$216
  Top 0.152: PC_AN4.2 109.27,55.35 109.27,57.3 110.16,58.19 114.61,58.19 116.74,56.06 116.74,52.68 117.09,52.32 117.09,49.12 117.8,48.41 117.8,42.37 115.49,40.06 113.18,40.06 112.47,39.34 112.47,38.63 BR_OR7.10
N$217
  Top 0.152: BR_OR6.1 107.85,43.79 105.36,41.3 105.36,37.92 109.8,33.48 109.8,32.59 BR_OR7.3
N$218  (via drill 0.35)
  Top 0.152: BR_OR1.5 31.75,44.68 33.71,46.63 v34.77,46.63 | v100.56,47.88 100.56,49.84 BR_JK2.10 | v100.2,15.34 109.8,15.34 112.29,17.83 112.29,18.36 BR_AN7.5 | v98.25,48.41 97.18,47.35 95.05,47.35 92.73,45.03 92.73,43.97 BR_JK2.1
  Route15 0.152: v34.77,46.63 34.77,47.17 43.48,55.88 92.2,55.88 96.65,51.44 97,51.44 v100.56,47.88
  Bottom 0.152: v100.2,15.34 100.56,15.7 v100.56,47.88 98.78,47.88 v98.25,48.41
N$219  (via drill 0.35)
  Top 0.152: BR_AN7.2 108.74,18.54 108.74,22.45 109.8,23.52 109.8,24.59 BR_AN7.12 109.98,24.77 109.98,26.19 v110.87,27.08 | v41.53,48.41 41,47.88 37.97,47.88 35.84,50.01 34.42,50.01 BR_OR1.8 | v92.91,48.41 93.98,49.48 BR_JK2.15
  Route2 0.152: v41.53,48.41 60.02,48.41 61.44,46.99 76.02,46.99 77.09,48.06 79.05,48.06 79.4,48.41 85.27,48.41 85.98,49.12 92.2,49.12 v92.91,48.41
  Route15 0.152: v110.87,27.08 103.23,34.72 103.23,36.14 92.91,46.46 v92.91,48.41
N$220
  Top 0.152: M_OR1.5 43.84,30.1 43.84,35.97 M_OR1.10
N$221
  Top 0.152: BR_OR6.2 109.09,43.97 109.09,45.92 106.25,48.77 106.25,50.72 109.45,53.92 109.63,53.92 110.34,54.63 110.34,55.35 PC_AN4.3
N$222  (via drill 0.35)
  Top 0.152: BR_AN7.1 107.31,22.81 108.56,24.05 108.56,24.59 BR_AN7.13 108.74,24.77 108.74,25.83 | 108.74,25.83 108.74,26.01 110.52,27.79 113.72,27.79 115.67,25.83 115.67,17.3 115.49,17.12 114.43,17.12 113.72,17.83 113.72,18.36 BR_AN7.6 | v108.03,80.24 107.31,80.95 107.31,81.66 107.85,82.19 107.85,84.33 PC_JK7.15 | 108.74,25.83 v108.03,26.54
  Bottom 0.152: v108.03,80.24 108.03,59.26 107.67,58.9 107.67,37.74 108.03,37.39 v108.03,26.54
N$223
  Top 0.152: M_OR1.4 42.42,29.92 42.42,29.21 40.28,27.08 38.68,27.08 37.97,26.37 37.97,23.52 38.68,22.81 38.68,18.54 PL_XR.1 38.86,18.36 38.86,17.83 40.82,15.88 46.33,15.88 47.04,16.59 47.04,17.48 49.53,19.96 52.55,19.96 53.26,19.25 53.26,18.54 M_NO1.3
N$224
  Top 0.152: 4.45,118.11 3.81,118.11 3.17,117.47 3.17,118.11 2.54,118.11 2.54,115.57 3.17,115.57 3.17,116.21 3.81,115.57 4.45,115.57 | 4.45,118.11 3.17,116.84 4.45,115.57 | 4.45,115.57 3.81,116.84 4.45,118.11
N$225
  Top 0.152: 22.86,115.57 22.86,118.11 23.49,118.11 24.77,116.21 24.77,118.11 25.4,118.11 25.4,115.57 24.77,115.57 23.49,117.47 23.49,115.57 22.86,115.57
N$226
  Top 0.152: 8.25,118.11 8.25,115.57 10.16,115.57 10.16,118.11 8.25,118.11
N$227
  Top 0.152: 8.89,117.47 8.89,116.21 9.53,116.21 9.53,117.47 8.89,117.47
N$228
  Top 0.152: 12.7,116.21 12.07,115.57 10.79,115.57 12.07,116.84 10.79,118.11 12.07,118.11 12.7,117.47 | 12.7,116.21 13.02,116.52 12.38,117.16 12.7,117.47 | 12.7,116.21 13.34,115.57 14.61,115.57 13.34,116.84 14.61,118.11 13.34,118.11 12.7,117.47
N$229
  Top 0.152: 5.71,117.47 5.71,115.57 5.08,115.57 5.08,118.11 5.71,118.11 6.99,116.21 6.99,118.11 7.62,118.11 7.62,115.57 6.99,115.57 5.71,117.47
N$230
  Top 0.152: 26.03,118.11 26.03,115.57 26.67,115.57 26.67,118.11 26.03,118.11
N$231
  Top 0.152: 27.3,118.11 27.3,115.57 27.94,115.57 arc90 28.58,116.21 arc90 27.94,116.84 arc90 28.58,117.47 arc90 27.94,118.11 27.3,118.11
N$232
  Top 0.152: 29.21,118.11 29.21,115.57 29.84,115.57 arc90 30.48,116.21 arc90 29.84,116.84 arc90 30.48,117.47 arc90 29.84,118.11 29.21,118.11
N$233
  Top 0.152: 31.12,118.11 31.12,115.57 32.38,115.57 32.38,116.21 31.75,116.21 31.75,118.11 31.12,118.11
N$234
  Top 0.152: 36.83,115.57 arc-180 36.83,118.11 36.83,117.47 arc180 36.83,116.21 36.83,115.57
N$235
  Top 0.152: 33.02,118.11 33.02,115.57 34.29,115.57 34.29,116.21 33.66,116.21 33.66,116.52 34.29,116.52 34.29,117.16 33.66,117.16 33.66,117.47 34.29,117.47 34.29,118.11 33.02,118.11
N$236
  Top 0.152: 37.46,118.11 37.46,115.57 38.1,115.57 38.1,116.84 arc90 38.73,117.47 arc90 38.1,118.11 37.46,118.11
N$237
  Top 0.152: 39.37,118.11 39.37,116.21 arc90 40,115.57 40.64,115.57 arc90 41.27,116.21 41.27,118.11 40.64,118.11 40.64,116.21 40,116.21 40,118.11 39.37,118.11
PC_N0  (via drill 0.35)
  Top 0.152: v105.36,81.31 106.6,80.06 106.6,78.28 PC_JK7.1
  Route2 0.152: v105.36,89.48 104.47,89.48 104.11,89.13 87.58,89.13 86.69,90.02 72.29,90.02 71.22,88.95 M48Z08.10
  Bottom 0.152: v105.36,89.48 v105.36,81.31
PC_N1  (via drill 0.35)
  Top 0.152: v103.76,95.53 105,94.28 107.14,94.28 107.85,95 107.85,95.71 PC_JK6.15
  Route2 0.152: v103.76,95.53 71.22,95.53 69.98,94.28 69.98,92.51 71.04,91.44 M48Z08.9
PC_N2  (via drill 0.35)
  Top 0.152: v104.83,90.37 105.54,90.37 106.25,89.66 106.6,89.66 PC_JK6.1
  Route2 0.152: v104.83,90.37 74.78,90.37 71.22,93.93 M48Z08.8
PC_N3  (via drill 0.35)
  Top 0.152: v100.38,104.06 100.74,104.42 106.25,104.42 107.85,106.02 107.85,107.09 PC_JK5.15 | v83.84,98.02 72.64,98.02 71.22,96.6 M48Z08.7
  Route15 0.152: v100.38,104.06 94.87,104.06 88.82,98.02 v83.84,98.02
PC_N4  (via drill 0.35)
  Top 0.152: v105.54,101.22 106.6,101.22 PC_JK5.1 | v83.49,100.15 72.29,100.15 71.22,99.09 M48Z08.6
  Route15 0.152: v105.54,101.22 104.29,101.22 100.74,104.78 93.98,104.78 92.91,103.71 89.89,103.71 86.33,100.15 v83.49,100.15
PC_N5  (via drill 0.35)
  Top 0.152: v117.45,73.84 116.74,74.55 108.91,74.55 108.03,73.66 108.03,72.95 PC_JK4.15
  Route2 0.152: v117.45,90.19 111.58,90.19 104.83,96.95 92.73,96.95 89.18,100.51 84.2,100.51 83.13,101.57 71.22,101.57 M48Z08.5
  Bottom 0.152: v117.45,90.19 v117.45,73.84
PC_N6  (via drill 0.35)
  Top 0.152: v106.6,69.57 106.6,66.9 PC_JK4.1 | v79.22,100.86 74.42,100.86 71.22,104.06 M48Z08.4
  Route15 0.152: v106.6,69.57 106.6,70.1 95.05,81.66 94.69,81.66 94.34,82.02 94.34,90.02 86.69,97.66 84.56,97.66 84.2,97.31 82.78,97.31 v79.22,100.86
PC_N7  (via drill 0.35)
  Top 0.152: PC_JK3.15 93.98,83.44 v93.27,82.73
  Route15 0.152: v93.27,82.73 93.27,83.44 86.33,90.37 85.62,90.37 72.11,103.89 72.11,105.66 71.22,106.55 M48Z08.3
PC_N8  (via drill 0.35)
  Top 0.152: v91.31,79.53 92.56,78.28 PC_JK3.1
  Bottom 0.152: v91.31,79.53 88.11,82.73 88.11,102.46 86.51,104.06 M48Z08.25
PC_N9
  Top 0.152: PC_JK2.15 93.98,96.42 88.82,101.57 86.51,101.57 M48Z08.24
PC_N10
  Top 0.152: PC_JK2.1 92.56,89.66 90.78,89.66 86.51,93.93 M48Z08.21
PC_N11
  Top 0.152: PC_JK1.15 93.98,104.78 93.62,104.42 88.29,104.42 87.58,105.13 80.82,105.13 79.22,103.53 79.22,102.82 79.58,102.46 82.96,102.46 M48Z08.23
PC_N12  (via drill 0.35)
  Top 0.152: v88.82,103.71 91.31,101.22 92.56,101.22 PC_JK1.1
  Route2 0.152: v88.82,103.71 88.29,103.71 86.33,105.66 74.78,105.66 71.22,109.22 M48Z08.2
SE_CLK  (via drill 0.35)
  Top 0.152: SE_JK6.13 13.97,95.17 13.08,94.28 12.37,94.28 | 12.37,94.28 9.7,94.28 9.35,94.64 9.35,98.37 10.59,99.62 11.84,99.62 12.55,100.33 12.55,101.04 SE_JK7.3 | v12.37,79.88 12.55,79.7 12.55,78.28 SE_JK5.3 | v12.37,82.73 12.9,82.73 13.97,83.8 SE_JK5.13 | v12.37,87.88 12.55,88.06 12.55,89.48 SE_JK6.3 | SE_JK7.13 13.97,106.02 14.15,105.84 14.15,105.13 13.79,104.78 v12.37,104.78 | v12.37,94.11 12.37,94.28 | v23.04,69.57 21.97,70.64 21.62,70.64 SE_CLK.2 | v23.04,66.02 24.28,66.02 24.99,65.3 27.13,65.3 27.84,66.02 27.84,66.73 SE_JK4.3 | v25.7,53.57 26.77,53.57 27.84,54.63 27.84,55.35 SE_JK3.3 28.02,55.35 28.02,56.59 29.44,58.01 31.93,58.01 v32.99,56.95 | v28.02,59.79 28.19,59.79 29.08,60.68 29.08,61.39 SE_JK3.13 | v27.48,71.17 28.02,71.17 29.08,72.24 29.08,72.77 SE_JK4.13 | v32.99,28.32 32.99,29.92 SE_AN3.6
  Route15 0.152: v12.37,79.88 12.72,79.88 v23.04,69.57
  Bottom 0.152: v12.37,79.88 v12.37,82.73 v12.37,87.88 v12.37,94.11 v12.37,104.78 | v23.04,69.57 v23.04,66.02 25.17,63.88 25.17,59.79 | v25.7,53.57 25.17,54.1 25.17,59.79 | 25.17,59.79 27.48,59.79 | 27.48,59.79 v28.02,59.79 | 27.48,59.79 v27.48,71.17 | v32.99,56.95 v32.99,28.32
SE_ENCLK  (via drill 0.35)
  Top 0.152: 16.28,66.9 16.46,66.9 SE_JK12.6 | 16.28,66.9 15.39,66.9 SE_JK12.5 | SE_JK12.10 17.7,72.95 16.64,72.95 SE_JK12.11 16.46,72.77 16.28,72.59 16.28,66.9 | 16.28,66.9 SE_JK12.6 | 27.66,22.28 27.3,22.63 24.1,22.63 18.24,28.5 17.35,28.5 16.64,29.21 16.64,29.92 SE_JK1.6 | 27.66,22.28 30.33,19.61 30.33,18.01 SE_N01.5 | SE_JK1.5 15.39,30.1 16.46,30.1 SE_JK1.6 | SE_AN3.10 31.75,36.68 30.68,37.74 v27.84,37.74 | 27.66,22.28 v27.84,22.28 | v17.35,65.13 16.64,65.84 16.64,66.73 SE_JK12.6 | v16.99,32.23 16.99,30.45 16.64,30.1 SE_JK1.6
  Bottom 0.152: v27.84,22.28 v27.84,37.74 | v17.35,65.13 17.35,34.54 17.17,34.37 17.17,32.41 v16.99,32.23
SE_N0  (via drill 0.35)
  Top 0.152: v67.31,114.02 66.42,114.91 66.06,114.91 SP_BF0.2 | v60.55,116.51 60.55,115.09 SEN0.1
  Bottom 0.152: M48Z08.11 71.04,86.46 69.44,88.06 69.44,111.89 v67.31,114.02 67.31,116.87 60.91,116.87 v60.55,116.51
SE_N1  (via drill 0.35)
  Top 0.152: v67.67,109.75 66.06,109.75 SP_BF1.2 | v61.27,111.35 60.73,110.82 60.73,109.93 SEN1.1
  Route2 0.152: v61.27,111.35 66.06,111.35 v67.67,109.75
  Bottom 0.152: v67.67,109.75 69.09,108.33 69.09,85.93 71.04,83.97 M48Z08.12
SE_N2  (via drill 0.35)
  Top 0.152: SEN2.1 60.73,104.78 61.09,104.42 62.69,104.42 63.04,104.78 SP_BF2.2 66.42,104.78 68.38,102.82 v68.38,101.22
  Bottom 0.152: v68.38,101.22 68.38,83.97 71.04,81.31 M48Z08.13
SE_N3  (via drill 0.35)
  Top 0.152: v59.84,96.42 62.51,96.42 64.47,98.37 64.47,98.55 65.53,99.62 65.89,99.62 SP_BF3.2 | v59.84,97.84 59.84,98.91 60.55,99.62 SEN3.1
  Route15 0.152: v59.84,96.42 61.62,96.42 70.16,87.88 72.47,87.88 74.24,86.11 74.24,82.37 76.2,80.42 82.42,80.42 84.02,78.82 86.33,78.82 M48Z08.15
  Bottom 0.152: v59.84,97.84 v59.84,96.42
SE_N4  (via drill 0.35)
  Top 0.152: SEN4.1 60.73,94.46 61.09,94.11 62.51,94.11 62.86,94.46 65.89,94.46 SP_BF4.2 66.06,94.46 67.49,94.46 68.2,93.75 68.2,92.15 69.98,90.37 72.29,90.37 74.07,88.59 82.6,88.59 82.96,88.95 v83.49,88.95
  Route2 0.152: M48Z08.16 83.67,83.97 83.67,88.77 v83.49,88.95
SE_N5
  Top 0.152: SEN5.2 60.73,89.66 65.89,89.66 SP_BF5.2 66.06,89.48 67.67,89.48 69.62,87.53 87.4,87.53 88.11,86.82 88.11,85.93 86.51,84.33 86.51,83.97 M48Z08.17
SE_N6
  Top 0.152: SEN6.2 60.73,84.51 65.89,84.51 SP_BF6.2 66.06,84.51 66.42,84.51 66.78,84.86 71.75,84.86 73.18,86.28 86.33,86.28 M48Z08.18
SE_N7
  Top 0.152: SP_BF7.2 65.89,79.53 60.73,79.53 SEN7.2 60.55,79.53 59.13,80.95 56.46,80.95 54.15,83.26 54.15,88.95 54.51,89.31 55.57,89.31 57.53,91.26 67.67,91.26 68.91,90.02 72.11,90.02 73.89,88.24 83.84,88.24 84.38,88.77 86.33,88.77 M48Z08.19
SE_NEWNUMBER  (via drill 0.35)
  Top 0.152: 17.7,103.53 15.75,103.53 13.97,101.75 SE_JK7.4 | 17.7,103.53 19.13,103.53 19.84,102.82 19.84,99.97 19.13,99.26 18.24,99.26 16.99,98.02 16.81,98.02 15.39,96.6 15.39,95.88 SE_JK6.12 | v17.7,109.75 16.1,109.75 15.39,109.04 15.39,107.26 SE_JK7.12 | 17.7,103.53 v17.7,104.42 | 13.97,77.57 SE_JK5.4 13.97,78.1 | 13.97,77.57 13.26,76.86 9.53,76.86 9.35,77.04 9.35,79.53 11.84,82.02 13.61,82.02 15.21,83.62 15.21,84.33 SE_JK5.12 15.21,84.51 15.21,85.04 14.33,85.93 v14.33,86.28 | SE_JK6.4 13.97,88.24 v14.33,87.88 | 25.17,69.22 22.33,66.37 22.33,60.68 19.66,58.01 14.68,58.01 13.97,57.3 SE_JK2.4 13.97,54.1 15.21,52.86 22.15,52.86 24.28,50.72 v25.7,50.72 | 25.17,69.22 27.48,69.22 29.08,67.62 29.08,66.9 SE_JK4.4 | 13.97,77.57 15.75,75.79 17.17,75.79 17.53,75.44 19.3,75.44 19.48,75.62 21.97,75.62 24.64,72.95 24.64,69.75 25.17,69.22 | v27.13,28.32 29.44,28.32 30.33,29.21 30.33,29.92 SE_AN3.4 | SE_JK3.4 29.08,55.35 29.08,54.63 28.19,53.75 v28.19,53.21 27.84,52.86 24.64,52.86 23.75,53.75 23.75,55.52 24.99,56.77 26.42,56.77 30.33,60.68 30.33,61.39 SE_JK3.12 30.33,61.57 30.15,61.75 30.15,64.06 30.86,64.77 v32.11,64.77 | v16.46,34.37 16.28,34.37 15.39,35.26 15.39,35.97 SE_JK1.12 | v32.11,70.64 30.51,72.24 30.51,72.77 SE_JK4.12 | v109.98,56.95 112.12,56.95 113,56.06 113,55.35 PC_AN4.5
  Route2 0.152: v16.46,34.37 22.5,28.32 v27.13,28.32
  Route15 0.152: v17.7,104.42 17.7,98.73 18.41,98.02 18.41,91.97 v14.33,87.88 | v109.98,56.95 108.03,56.95 107.31,56.24 106.25,56.24 105.54,56.95 99.14,56.95 98.42,56.24 31.22,56.24 v28.19,53.21
  Bottom 0.152: v17.7,104.42 v17.7,109.75 | v14.33,86.28 v14.33,87.88 | 27.13,50.72 27.13,52.15 v28.19,53.21 | 27.13,50.72 v27.13,28.32 | v32.11,64.77 v32.11,70.64 | 27.13,50.72 v25.7,50.72
SE_WRITE_N  (via drill 0.35)
  Top 0.152: PC_AN1.9 129.54,59.08 | 129.54,59.08 PC_AN1.6 | v123.85,56.95 124.38,56.41 124.38,55.35 PC_AN1.2 | v123.85,59.79 123.85,60.86 124.38,61.39 PC_AN1.13 | v123.85,59.79 123.14,59.08 122.43,59.08 120.12,61.39 115.67,61.39 PC_AN4.8 | 129.54,59.08 124.56,59.08 v123.85,59.79 | 93.98,67.44 93.27,68.15 87.05,68.15 86.51,67.62 86.51,66.9 PC_AN2.6 | 93.98,67.44 PC_AN3.2 93.98,66.9 | 99.14,68.68 99.14,68.86 98.78,69.22 95.76,69.22 93.98,67.44 | 99.14,68.68 99.14,66.9 PC_AN3.6 | v100.02,71.17 99.14,72.06 99.14,72.77 PC_AN3.9 | 99.14,68.68 v99.67,68.68 | v109.8,59.79 109.27,60.33 109.27,61.39 PC_AN4.13 | SP_BF0.1 65.89,113.84 64.47,112.42 64.47,110.11 65.53,109.04 65.89,109.04 SP_BF1.1 66.06,109.04 67.31,109.04 | 67.31,109.04 68.02,109.04 68.38,109.4 68.38,111.71 70.33,113.66 86.69,113.66 88.11,112.24 88.11,111.35 86.51,109.75 86.51,109.22 M48Z08.27 | v81.18,68.5 81.18,66.9 PC_AN2.2 | PC_AN2.13 81.18,72.95 v81.18,74.55 82.6,75.97 85.27,75.97 86.33,74.91 86.33,72.95 PC_AN2.9 | 67.13,79.17 66.42,78.46 66.06,78.46 SP_BF7.1 | 67.13,79.17 67.13,82.37 66.78,82.73 | 66.78,82.73 66.06,83.44 SP_BF6.1 | v66.95,87.53 66.06,88.42 SP_BF5.1 | 66.78,82.73 v66.95,82.73 | v66.95,92.69 66.06,93.57 SP_BF4.1 | v66.95,97.84 66.06,98.73 SP_BF3.1 | v66.95,102.82 66.06,103.71 SP_BF2.1 | v20.55,62.99 20.19,63.35 13.97,63.35 12.72,62.1 12.72,61.57 SE_JK2.14 | PC_AN3.13 93.98,73.48 89.71,77.75 81.18,77.75 | 81.18,77.75 68.56,77.75 67.13,79.17 | 81.18,77.75 v81.18,78.1 | v67.31,108.69 67.31,109.04
  Route2 0.152: v20.55,62.99 47.93,62.99 66.95,82.02 v66.95,82.73
  Route15 0.152: v100.02,71.17 100.74,70.46 100.74,68.33 109.27,59.79 v109.8,59.79 110.52,59.08 113.54,59.08 115.32,57.3 121.54,57.3 122.96,58.73 122.96,58.9 v123.85,59.79 | v99.67,68.68 99.31,68.68 94.16,73.84 84.91,73.84 84.2,74.55 v81.18,74.55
